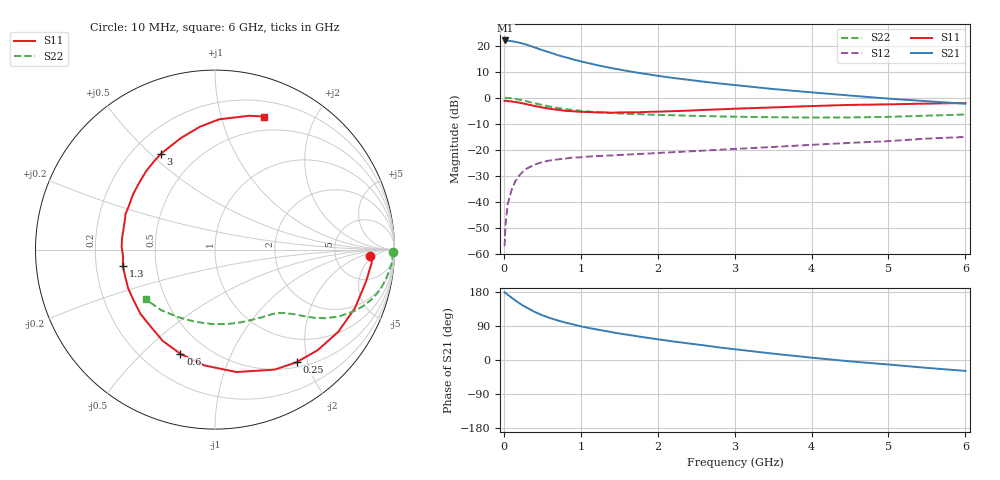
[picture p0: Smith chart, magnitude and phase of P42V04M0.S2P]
! SIEMENS Small Signal Semiconductors
! BFP182
! Si NPN RF Bipolar Junction Transistor in SOT143
! VCE = 2 V  IC = 4 mA
! Common Emitter S-Parameters:  March  1996
# GHz  S  MA  R  50
!  f  S11  S21  S12  S22
! GHz  MAG  ANG  MAG  ANG  MAG  ANG  MAG  ANG
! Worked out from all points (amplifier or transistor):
!   36 points, 10 MHz to 6 GHz, reference 50 ohm
!   highest |S21| = 22.0 dB at 20 MHz (marker M1)
!   |S21| within 3 dB of that: start of sweep to 431.7 MHz
!   unconditionally stable (mu >= 1): 1.69 GHz to 5.677 GHz
!   at 250 MHz: K = 0.19, MSG = 24.6 dB, |S12| = -28.4 dB
!   at 1.4 GHz: K = 0.89, MSG = 16.8 dB, |S12| = -22.2 dB
!   at 6 GHz: K = 0.96, MSG = 6.4 dB, |S12| = -15.1 dB
!   S11 on the Smith chart (normalised r, x): 10 MHz: 13, -4; 250 MHz: 0.58, -1.82; 600 MHz: 0.36, -0.66; 1.3 GHz: 0.32, -0.08; 3 GHz: 0.32, +0.54; 6 GHz: 0.35, +1.38
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0.01  0.8669 -2.4  12.5 178.6  0.0014 78.7  0.9924 -0.9
0.02  0.8764 -4.7  12.58 177.3  0.0033 89.8  0.9911 -1.8
0.05  0.8608 -11.6  12.46 172.2  0.009 87.8  0.9874 -4.6
0.1  0.8455 -22.5  12.21 164.6  0.0167 76.7  0.9689 -9.2
0.15  0.8255 -33.7  11.81 157.2  0.025 71.4  0.9481 -13.5
0.2  0.8007 -44.4  11.46 150.1  0.0319 67.1  0.9189 -17.3
0.25  0.7751 -54.0  10.9 143.5  0.038 61.7  0.8845 -20.8
0.3  0.7465 -63.6  10.4 138.0  0.0436 57.4  0.8488 -23.8
0.4  0.6924 -80.1  9.253 127.0  0.0517 50.6  0.7837 -28.4
0.5  0.6477 -95.4  8.208 118.1  0.058 44.7  0.7253 -31.8
0.6  0.6117 -108.4  7.393 110.7  0.0622 40.9  0.6746 -34.3
0.7  0.5864 -119.7  6.573 104.4  0.0651 37.8  0.6355 -36.1
0.8  0.5588 -129.9  5.983 98.7  0.0676 35.3  0.6039 -37.5
1.1  0.5298 -156.0  4.616 84.6  0.074 30.7  0.5428 -41.0
1.3  0.522 -169.7  3.961 77.2  0.0766 29.3  0.5162 -43.1
1.7  0.5222 167.7  3.084 63.8  0.082 28.3  0.4839 -47.8
2.2  0.5505 146.1  2.394 49.0  0.0895 27.7  0.4602 -55.0
3  0.6134 119.3  1.75 28.4  0.1035 27.1  0.4313 -69.6
3.5  0.6502 106.9  1.467 16.8  0.1131 25.9  0.4207 -80.5
4.5  0.7262 88.2  1.099 -3.6  0.1351 22.6  0.4172 -105.4
5.5  0.77 75.6  0.856 -20.8  0.1635 18.2  0.4511 -131.5
6  0.7902 69.7  0.763 -28.8  0.1758 14.1  0.4751 -144.2
